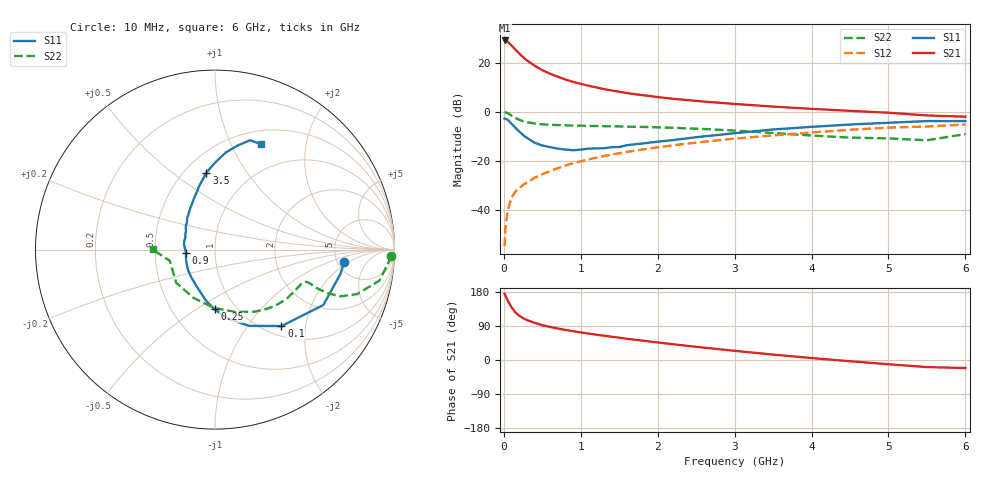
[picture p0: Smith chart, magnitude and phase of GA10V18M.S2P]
! Infineon Technologies  Discrete & RF Semiconductors
! BF775
! Si NPN RF Bipolar Junction Transistor in SOT23
! VCE = 10 V  IC = 18 mA
! Common Emitter S-Parameters:  May  1996
# GHz  S  MA  R  50
!  f  S11  S21  S12  S22
! GHz  MAG  ANG  MAG  ANG  MAG  ANG  MAG  ANG
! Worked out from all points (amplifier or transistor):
!   36 points, 10 MHz to 6 GHz, reference 50 ohm
!   highest |S21| = 29.0 dB at 10 MHz (marker M1)
!   |S21| within 3 dB of that: start of sweep to 128.1 MHz
!   unconditionally stable (mu >= 1): 475.9 MHz to 2.683 GHz
!   at 250 MHz: K = 0.79, MSG = 26.0 dB, |S12| = -29.9 dB
!   at 1.4 GHz: K = 1.09, MAG = 11.2 dB, |S12| = -17.5 dB
!   at 6 GHz: K = 0.88, MSG = 1.6 dB, |S12| = -5.3 dB
!   S11 on the Smith chart (normalised r, x): 10 MHz: 5.74, -1.63; 100 MHz: 1.18, -1.47; 250 MHz: 0.80, -0.60; 900 MHz: 0.72, -0.03; 3.5 GHz: 0.63, +0.67; 6 GHz: 0.65, +1.30
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0.01  0.7228 -5.4  28.23 174.6  0.0018 91.1  0.9824 -2.1
0.02  0.712 -11.0  27.7 169.9  0.0042 83.9  0.9677 -4.5
0.05  0.678 -27.1  26.48 157.0  0.0097 78.3  0.9319 -10.7
0.1  0.5644 -49.0  22.36 139.2  0.0176 71.3  0.8298 -17.4
0.15  0.4656 -65.9  18.31 125.8  0.0234 66.2  0.7437 -20.5
0.2  0.3914 -79.5  15.27 117.0  0.0274 65.4  0.6796 -21.1
0.25  0.3328 -90.4  12.83 110.4  0.0319 65.4  0.6356 -21.0
0.3  0.2908 -99.5  11.07 105.3  0.0358 66.7  0.6069 -20.7
0.4  0.2317 -115.6  8.626 98.1  0.0447 67.7  0.5718 -19.9
0.5  0.2031 -130.7  7.004 91.9  0.0528 68.9  0.5499 -19.4
0.6  0.1885 -142.5  5.934 87.3  0.0614 69.2  0.5383 -19.5
0.7  0.176 -154.3  5.143 83.1  0.0701 69.9  0.5302 -20.0
0.9  0.1627 -173.6  4.041 75.9  0.0885 69.3  0.5186 -21.3
1.1  0.1755 170.2  3.375 69.9  0.1058 68.9  0.511 -23.6
1.3  0.1786 157.2  2.882 64.2  0.1241 67.5  0.504 -26.0
1.6  0.2062 142.4  2.389 56.0  0.1508 65.4  0.4928 -30.2
2.2  0.2623 122.5  1.822 41.6  0.2051 60.4  0.4664 -40.2
2.6  0.313 111.5  1.598 32.6  0.2424 56.7  0.4409 -48.1
3.5  0.4319 96.4  1.264 14.3  0.3273 46.9  0.3659 -71.8
4.5  0.5448 83.6  1.037 -3.3  0.4256 34.7  0.2946 -113.9
5.5  0.6402 72.2  0.835 -18.7  0.4967 19.1  0.2598 -166.2
6  0.6406 66.6  0.786 -21.2  0.5459 14.9  0.348 179.9
